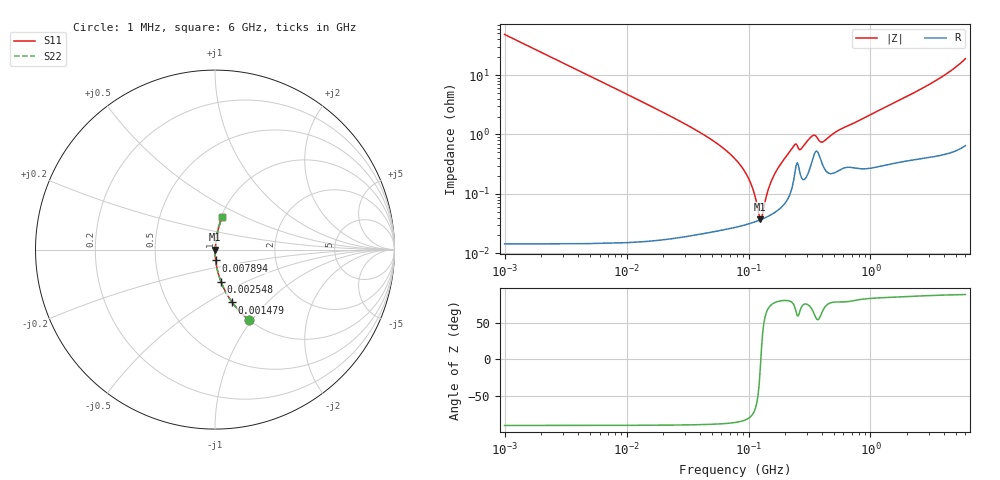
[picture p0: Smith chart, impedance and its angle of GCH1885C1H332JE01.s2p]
!Murata Part Number: GCH1885C1H332JE01
!These Parameters are Measured in Series Mode Connection
!Data Generated on Jun 19, 2026
!  o--ll--o
!Port1  Port2
!  o------o
!Operation Temp=25[degC], DC Bias Voltage=0[V]
!Freq. Start=1000[kHz] Stop=6[GHz] 401[Steps]
# Hz S RI R 50
!Freq.(Hz) S11(Real) S11(Imag) S21(Real) S21(Imag) S12(Real) S12(Imag) S22(Real) S22(Imag)
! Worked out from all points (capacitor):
!   401 points, 1 MHz to 6 GHz, reference 50 ohm
!   read as one part in series: C = 3.31 nF near 1.044 MHz
!   lowest |Z| = 37.3 mohm at 125 MHz (marker M1)
!   series resonance near 126.1 MHz, so ESL is about 480 pH
!   S11 on the Smith chart (normalised r, x): 1 MHz: 1.00, -0.96; 1.479 MHz: 1.00, -0.65; 2.548 MHz: 1.00, -0.38; 7.894 MHz: 1.00, -0.12; 6 GHz: 1.01, +0.38
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1000000  0.1882 -0.3907  0.8118 0.3907  0.8118 0.3907  0.1882 -0.3907
1479166  0.0959 -0.2942  0.9041 0.2942  0.9041 0.2942  0.0959 -0.2942
2547717  0.0346 -0.1823  0.9654 0.1823  0.9654 0.1823  0.0346 -0.1823
4293785  0.0125 -0.1106  0.9875 0.1106  0.9875 0.1106  0.0125 -0.1106
7894251  0.00382 -0.0605  0.9962 0.0605  0.9962 0.0605  0.00382 -0.0605
1.843659e7  0.000817 -0.0255  0.9992 0.0255  0.9992 0.0255  0.000817 -0.0255
4.697123e7  0.0003 -0.00881  0.9997 0.00881  0.9997 0.00881  0.0003 -0.00881
7.745967e7  0.000288 -0.00388  0.9997 0.00388  0.9997 0.00388  0.000288 -0.00388
9.019724e7  0.000301 -0.00262  0.9997 0.00262  0.9997 0.00262  0.000301 -0.00262
1.027698e8  0.00032 -0.00159  0.9997 0.00159  0.9997 0.00159  0.00032 -0.00159
1.249896e8  0.000366 -7.08e-05  0.9996 7.08e-05  0.9996 7.08e-05  0.000366 -7.08e-05
1.305463e8  0.00038 0.000268  0.9996 -0.000268  0.9996 -0.000268  0.00038 0.000268
1.520136e8  0.000445 0.00148  0.9996 -0.00148  0.9996 -0.00148  0.000445 0.00148
1.809028e8  0.000575 0.00299  0.9994 -0.00299  0.9994 -0.00299  0.000575 0.00299
2.348496e8  0.00177 0.00614  0.9982 -0.00614  0.9982 -0.00614  0.00177 0.00614
2.675853e8  0.00207 0.0052  0.9979 -0.0052  0.9979 -0.0052  0.00207 0.0052
3.325952e8  0.00367 0.00864  0.9963 -0.00864  0.9963 -0.00864  0.00367 0.00864
4.133993e8  0.00285 0.00709  0.9971 -0.00709  0.9971 -0.00709  0.00285 0.00709
5.60538e8  0.00266 0.0118  0.9973 -0.0118  0.9973 -0.0118  0.00266 0.0118
1.428092e9  0.00408 0.0307  0.9959 -0.0307  0.9959 -0.0307  0.00408 0.0307
3.408564e9  0.0105 0.0787  0.9895 -0.0787  0.9895 -0.0787  0.0105 0.0787
6e9  0.0401 0.1797  0.9599 -0.1797  0.9599 -0.1797  0.0401 0.1797
